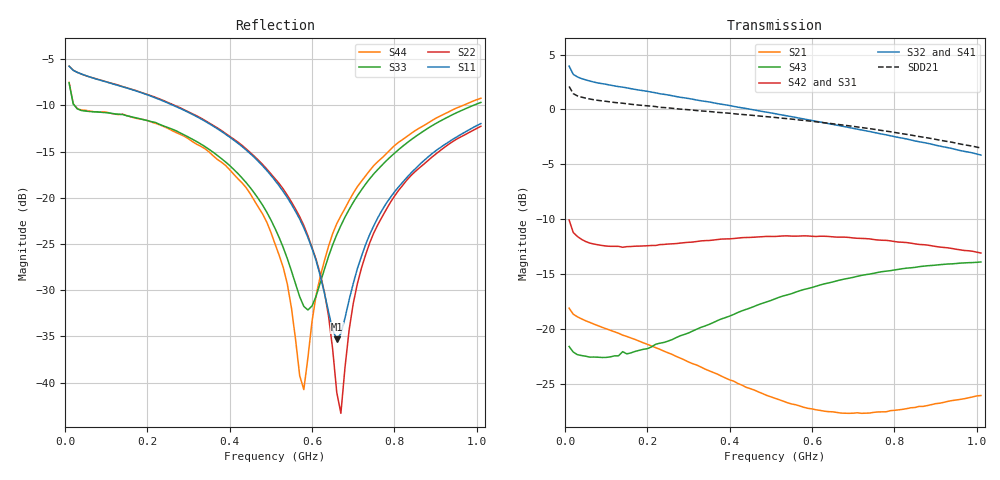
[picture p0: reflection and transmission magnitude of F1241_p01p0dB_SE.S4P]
! Integrated Device Technology
! Corporate Headquarters
! 6024 Silver Creek Valley Road
! San Jose, CA 95138  USA
! Phone:  1-408-284-8200
! Toll Free:  1-800-223-1366
! Webpage:  http://www.idt.com/
! Timing and RF Division
! 515 Groton Road, Suite 102
! Westford, MA 01886-6024
! Device:  F1241
! Description: Dual Intermediate Frequency Digital Variable Gain Amplifier
! Frequency:  10.0 -  500.00 MHz
! Package:  5x5 mm QFN Plastic Package: 32 pin
! Ports:  8 RF, 20 DC
!  Pin  1  = GA3  Pin 17  = RF OUT_B+
!  Pin  2  = GA4  Pin 18  = RF OUT_B-
!  Pin  3  = GA5  Pin 19  = STBY_B
!  Pin  4  = ISET_A  Pin 20  = Ground
!  Pin  5  = ISET_B  Pin 21  = Ground
!  Pin  6  = GB5  Pin 22  = STB_A
!  Pin  7  = GB4  Pin 23  = RF OUT_A-  = Port 4
!  Pin  8  = GB3  Pin 24  = RF OUT_A+  = Port 3
!  Pin  9  = GB2  Pin 25  = NO CONNECT
!  Pin 10  = GB1  Pin 26  = NO CONNECT
!  Pin 11  = RF IN_B+  Pin 27  = VCC
!  Pin 12  = RF IN_B-  Pin 28  = Ground
!  Pin 13  = Ground  Pin 29  = RF IN_A-  = Port 2
!  Pin 14  = VCC  Pin 30  = RF IN_A+  = Port 1
!  Pin 15  = NO CONNECT  Pin 31  = GA1
!  Pin 16  = NO CONNECT  Pin 32  = GA2
! State:  19
! Gain State:  1.0 dB
! Voltages:  Vcc = +5.00 Volts  Icc approximately 160.0 mA or 80 mA per channel.
! Data:  The device was measured on a custom evaluation board which has
!  individual transmission lines to the RF pins.  Data was collected
!  using a calibrated network analyzer.  The evaluation board was
!  de-embedded using a port reference technique.
!  The reference plane is the edge of the package pin.
!  Only Channel A was measured.
!  This data is in single-ended operation.  If your needs are balanced
!  or differential S-parameters then this file needs to be used a
!  linear simulator.
! Misc:  Lot Code  160028MY
!  Action Tracker AT004
! Date Measured:  2014-08-14
! Date:  2014-08-28  MJV
! Note:
!  Integrated Device Technology supplies this data as a sample of measured
!  data at the package pin for this product.  Your particular data for this
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# Hz S dB R 50
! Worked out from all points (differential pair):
!   101 points, 10 MHz to 1.01 GHz, reference 50 ohm
!   strongest paths, dB at 10 MHz, 260 MHz, 510 MHz, 760 MHz, 1.01 GHz:
!     S32: 3.9, 1.2, -0.4, -2.2, -4.2
!     S41: 4.0, 1.2, -0.5, -2.3, -4.4
!     S42: -10.1, -12.3, -11.6, -11.9, -13.1
!     S31: -10.1, -12.3, -11.6, -12.0, -13.2
!     S43: -21.6, -21.0, -17.3, -14.9, -13.9
!     S21: -18.1, -22.3, -26.3, -27.6, -26.1
!   taken as a pair (ports 2,1 in; 3,4 out), SDD21 dB: 2.1, 0.1, -0.7, -1.9, -3.5
!   lowest |S11| = -35.3 dB at 660 MHz (marker M1), VSWR 1.03, Z = 48.9 - j1.25 ohm
!   |S11| at or under -10 dB: 262.4 MHz to end of sweep
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1e7  -5.77 -11.2  -18.11 -15.4  -36.49 0.5  -20.91 10.6
     -18.12 -15.4  -5.77 -11.0  -20.93 10.4  -36.57 0.7
     -10.08 159.2  3.94 171.1  -7.59 -34.6  -21.68 -176.6
     3.97 171.2  -10.09 159.3  -21.62 -176.6  -7.52 -34.5
4.4e8  -14.84 -41.9  -25.23 -30.7  -33.53 16.6  -21.69 -26.6
       -25.34 -31.2  -14.72 -37.7  -21.53 -26.1  -33.48 15.0
       -11.75 44.2  0.07 113.7  -18.37 -39.3  -18.44 103.8
       0.01 112.6  -11.68 43.5  -18.23 103.3  -18.92 -35.1
5.3e8  -19.33 -50.2  -26.43 -26.3  -32.48 14.5  -21.69 -32.4
       -26.60 -27.0  -19.06 -43.6  -21.46 -31.9  -32.48 12.0
       -11.64 26.4  -0.53 102.9  -25.39 -59.7  -17.24 90.7
       -0.62 101.7  -11.54 25.5  -17.01 90.3  -27.54 -47.9
5.8e8  -23.25 -58.0  -26.92 -22.7  -31.99 12.4  -21.71 -35.7
       -27.16 -23.4  -23.00 -47.5  -21.44 -35.3  -31.99 10.1
       -11.64 17.3  -0.88 97.1  -31.75 -108.3  -16.67 83.7
       -0.98 95.9  -11.53 16.2  -16.42 83.3  -40.75 -132.0
6.6e8  -35.33 -131.9  -27.36 -16.3  -31.24 9.1  -21.80 -41.2
       -27.63 -16.2  -41.07 -93.1  -21.46 -40.8  -31.21 6.7
       -11.75 3.9  -1.44 88.2  -23.99 162.3  -15.85 72.9
       -1.57 86.8  -11.65 2.5  -15.64 72.7  -22.81 145.8
7.6e8  -22.14 141.3  -27.37 -8.6  -30.42 4.0  -22.01 -48.1
       -27.59 -7.9  -22.90 136.0  -21.56 -47.9  -30.36 1.2
       -12.03 -11.2  -2.18 77.4  -16.94 144.3  -15.09 60.0
       -2.35 76.0  -11.91 -13.1  -14.86 59.8  -16.08 136.4
1.01e9  -11.98 124.0  -26.05 1.4  -28.87 -11.3  -22.94 -64.2
        -26.09 3.0  -12.27 123.7  -22.24 -64.3  -28.83 -14.6
        -13.24 -41.2  -4.17 52.7  -9.69 127.7  -14.15 32.0
        -4.41 51.6  -13.09 -44.4  -13.91 31.8  -9.24 123.7
